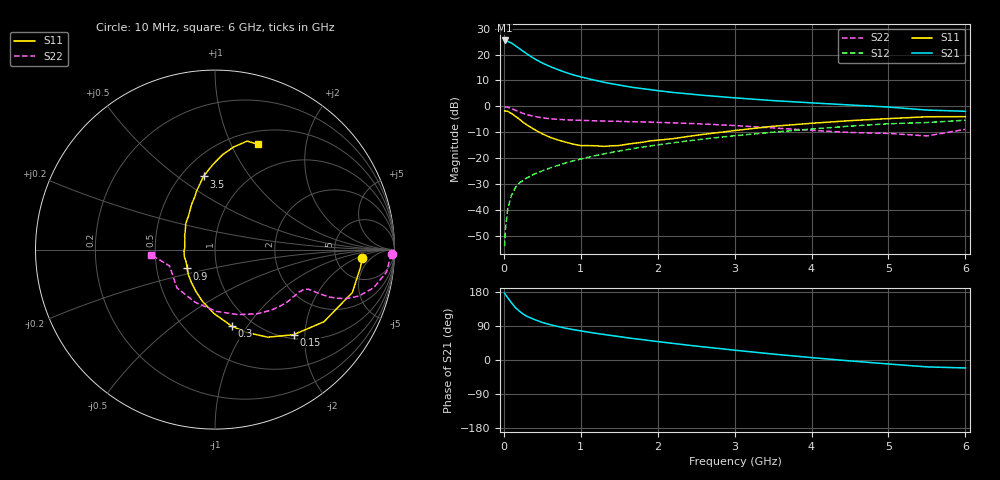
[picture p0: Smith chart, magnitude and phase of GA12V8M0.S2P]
! Infineon Technologies  Discrete & RF Semiconductors
! BF775
! Si NPN RF Bipolar Junction Transistor in SOT23
! VCE = 12 V  IC = 8 mA
! Common Emitter S-Parameters:  May  1996
# GHz  S  MA  R  50
!  f  S11  S21  S12  S22
! GHz  MAG  ANG  MAG  ANG  MAG  ANG  MAG  ANG
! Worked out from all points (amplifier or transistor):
!   36 points, 10 MHz to 6 GHz, reference 50 ohm
!   highest |S21| = 25.5 dB at 10 MHz (marker M1)
!   |S21| within 3 dB of that: start of sweep to 196.3 MHz
!   unconditionally stable (mu >= 1): 724.8 MHz to 2.799 GHz
!   at 250 MHz: K = 0.59, MSG = 24.9 dB, |S12| = -28.6 dB
!   at 1.4 GHz: K = 1.09, MAG = 11.4 dB, |S12| = -17.8 dB
!   at 6 GHz: K = 0.87, MSG = 1.7 dB, |S12| = -5.3 dB
!   S11 on the Smith chart (normalised r, x): 10 MHz: 9.37, -2.82; 150 MHz: 1.08, -1.75; 300 MHz: 0.81, -0.85; 900 MHz: 0.72, -0.16; 3.5 GHz: 0.64, +0.63; 6 GHz: 0.65, +1.27
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0.01  0.8219 -3.4  18.74 176.1  0.002 78.8  0.9889 -1.5
0.02  0.8161 -7.1  18.6 172.9  0.0041 78.9  0.9758 -3.0
0.05  0.8016 -17.4  18 164.4  0.0103 79.6  0.9647 -7.4
0.1  0.728 -33.5  16.7 150.7  0.0194 73.8  0.9095 -13.5
0.15  0.6452 -47.3  14.85 138.3  0.0271 68.0  0.8423 -17.9
0.2  0.5698 -58.9  13.15 129.3  0.033 64.5  0.7844 -20.3
0.25  0.4937 -69.2  11.65 121.3  0.0373 62.5  0.7311 -21.8
0.3  0.4376 -77.5  10.31 115.3  0.0416 62.8  0.6899 -22.5
0.4  0.3554 -91.1  8.298 106.7  0.0498 61.6  0.6374 -22.9
0.5  0.2953 -104.0  6.866 99.1  0.0569 62.3  0.6008 -22.9
0.6  0.2532 -115.5  5.896 93.4  0.0646 63.0  0.5774 -22.9
0.7  0.2254 -125.8  5.144 88.5  0.0723 64.0  0.5627 -23.1
0.9  0.187 -145.9  4.069 80.3  0.0887 64.1  0.5434 -24.1
1.1  0.1753 -166.3  3.417 73.6  0.1046 64.1  0.5311 -25.9
1.3  0.1685 176.0  2.923 67.4  0.1212 64.0  0.5208 -27.7
1.6  0.1856 155.6  2.428 58.8  0.1463 62.8  0.508 -31.4
2.2  0.2383 128.4  1.858 43.8  0.1982 59.1  0.4809 -40.7
2.8  0.3136 111.1  1.546 30.3  0.2528 53.9  0.4408 -52.3
3.5  0.4128 98.9  1.293 15.7  0.3172 46.8  0.3839 -70.6
4.5  0.5302 85.5  1.064 -2.4  0.4158 35.1  0.3137 -110.5
5.5  0.6303 73.5  0.849 -18.2  0.4879 20.0  0.269 -160.2
6  0.6343 67.7  0.804 -21.0  0.5405 15.8  0.3597 -175.6
